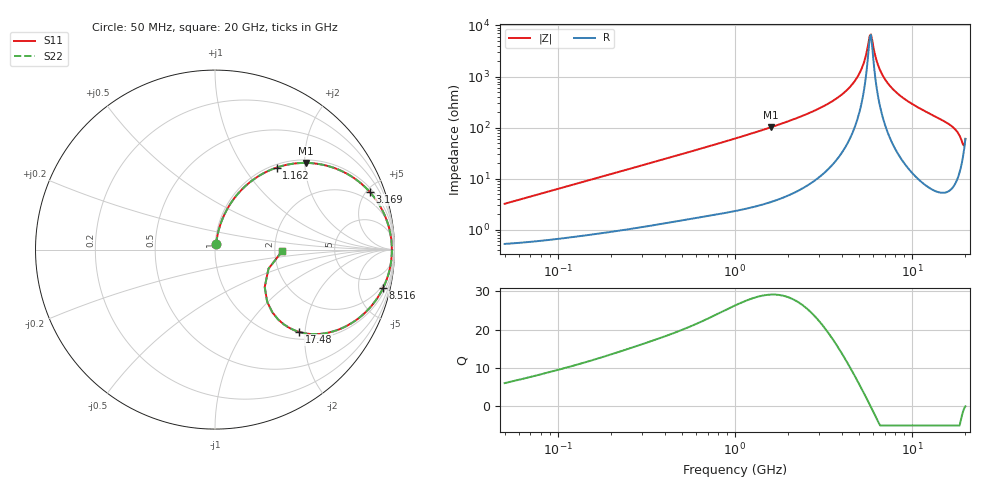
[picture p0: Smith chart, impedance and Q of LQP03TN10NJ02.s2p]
!Murata Part Number: LQP03TN10NJ02
!These Parameters are Measured in Series Mode Connection
!  o--[Z]--o
!Port1  Port2
!  o-------o
!Freq. Start=50[MHz] Stop=20[GHz], 401[Steps]
# Hz S RI R 50
!Freq.(Hz) S11(Real) S11(Imag) S21(Real) S21(Imag) S12(Real) S12(Imag) S22(Real) S22(Imag)
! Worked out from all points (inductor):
!   401 points, 50 MHz to 20 GHz, reference 50 ohm
!   read as one part in series: L = 10.1 nH near 51.52 MHz
!   highest Q = 29.1 at 1.591 GHz (marker M1), where L = 10.1 nH
!   self-resonance near 5.769 GHz
!   S11 on the Smith chart (normalised r, x): 50 MHz: 1.01, +0.06; 1.162 GHz: 1.05, +1.43; 3.169 GHz: 1.25, +5.27; 8.516 GHz: 1.54, -8.56; 17.48 GHz: 1.16, -1.86; 20 GHz: 2.20, -0.03
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5e7  0.00625 0.0315  0.9937 -0.0315  0.9937 -0.0315  0.00625 0.0315
1.364002e8  0.0145 0.0831  0.9855 -0.0831  0.9855 -0.0831  0.0145 0.0831
3.721004e8  0.0595 0.21  0.9405 -0.21  0.9405 -0.21  0.0595 0.21
1e9  0.2791 0.4299  0.7209 -0.4299  0.7209 -0.4299  0.2791 0.4299
1.161586e9  0.3439 0.4572  0.6561 -0.4572  0.6561 -0.4572  0.3439 0.4572
1.590961e9  0.5064 0.4831  0.4936 -0.4831  0.4936 -0.4831  0.5064 0.4831
2.728004e9  0.7981 0.3812  0.2019 -0.3812  0.2019 -0.3812  0.7981 0.3812
3.168813e9  0.8627 0.3209  0.1373 -0.3209  0.1373 -0.3209  0.8627 0.3209
4.026975e9  0.9394 0.2048  0.0606 -0.2048  0.0606 -0.2048  0.9394 0.2048
4.748272e9  0.9711 0.1158  0.0289 -0.1158  0.0289 -0.1158  0.9711 0.1158
5.194772e9  0.9808 0.0654  0.0192 -0.0654  0.0192 -0.0654  0.9808 0.0654
5.433528e9  0.9837 0.0399  0.0163 -0.0399  0.0163 -0.0399  0.9837 0.0399
5.683258e9  0.9852 0.0143  0.0148 -0.0143  0.0148 -0.0143  0.9852 0.0143
5.856089e9  0.9855 -0.00288  0.0145 0.00288  0.0145 0.00288  0.9855 -0.00288
6.503449e9  0.9816 -0.063  0.0184 0.063  0.0184 0.063  0.9816 -0.063
7.442007e9  0.9655 -0.1398  0.0345 0.1398  0.0345 0.1398  0.9655 -0.1398
8.516016e9  0.9363 -0.2146  0.0637 0.2146  0.0637 0.2146  0.9363 -0.2146
1.314879e10  0.7439 -0.4196  0.2561 0.4196  0.2561 0.4196  0.7439 -0.4196
1.747767e10  0.4678 -0.4585  0.5322 0.4585  0.5322 0.4585  0.4678 -0.4585
1.855685e10  0.3515 -0.389  0.6485 0.389  0.6485 0.389  0.3515 -0.389
1.912117e10  0.2904 -0.29  0.7096 0.29  0.7096 0.29  0.2904 -0.29
2e10  0.3759 -0.00628  0.6241 0.00628  0.6241 0.00628  0.3759 -0.00628
